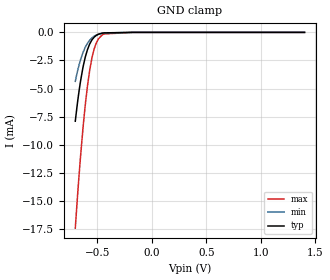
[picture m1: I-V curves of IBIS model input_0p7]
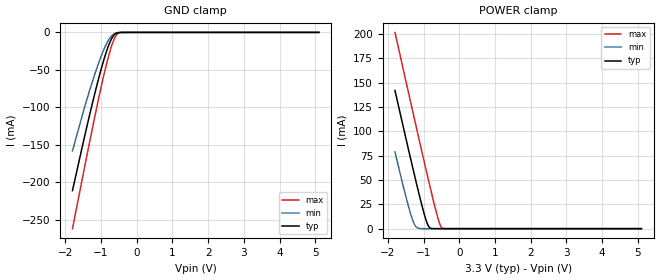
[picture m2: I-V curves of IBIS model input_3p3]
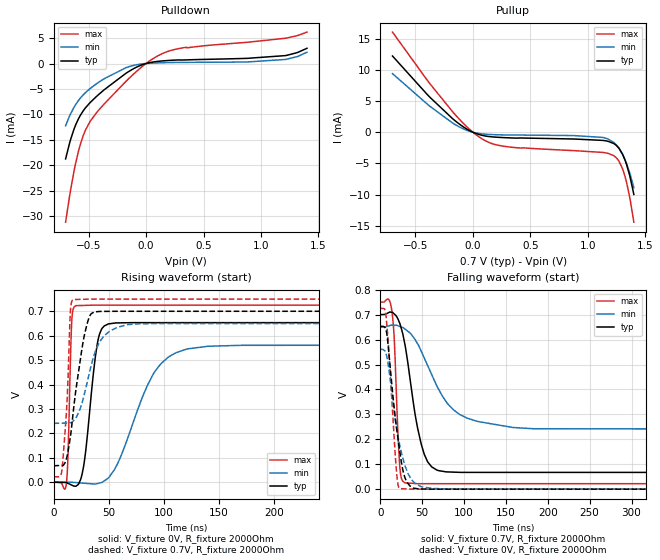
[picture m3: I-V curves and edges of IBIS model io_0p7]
|Texas Instruments Incorporated
| SN74AXCH8T245 8-Bit Dual-Supply Bus Transceiver with Configurable Voltage
| Translation, Tri-State Outputs, and Bus-Hold Circuitry
[IBIS Ver]   4.1
[File name]   sn74axch8t245.ibs
[Date]   01/24/2019
[File Rev]   2.0
[Source]
| Texas Instruments Incorporated.
| Analog-eLab Design Center, HPA
| 12500 TI Blvd
| Dallas, TX -75243
[Notes]
| Rev 2.0: 01/24/2019
| - Added SN74AXCH8T245RHL component
| Rev 1.0: 08/07/2018
| - Initial version of the model
| - Model generated from simulations in SPECTRE
| - Warnings regarding combined Non-monotonicity of various models
|   have been reviewed and considered minor and can be ignored.
| - C_comp although listed in numerical order of value are
|   obtained from varying PVT conditions. For PVT conditions for
|   each specific value refer the buffer description under
|   respective [Model]. IBIS model user is responsible for using
|   appropriate C_comp to simulate for Signal Integrity.
[Disclaimer]
| This model is designed as an aid for customers of Texas Instruments.
| TI and its licensors and suppliers make no warranties, either expressed
| or implied, with respect to this  model, including the warranties of
| merchantability or fitness for a particular purpose. The model is
| provided solely on an "as is" basis. The entire risk as to its quality
| and performance is with the customer.
| This model is subject to change without notice. Texas Instruments
| Incorporated is not responsible for updating this model.
[Copyright]
(C) Copyright 2019 Texas Instruments Incorporated.All rights reserved.
|  Component SN74AXCH8T245PW 24-pin TSSOP - PW package
|  Part # SN74AXCH8T245PW
[Component]   SN74AXCH8T245PW
[Manufacturer]  TI
[Package]   |24 TSSOP - PW package
|   typ   min   max
R_pkg   0.1143375   0.06811   0.12769
L_pkg   3.405334167nH   2.85598nH   4.17092nH
C_pkg   0.565412083pF   0.46044pF   0.71557pF
[Pin]  signal_name model_name  R_pin   L_pin   C_pin
1   VCCA   power   0.06958   3.86966nH   0.71557pF
2   DIR1   input   0.12094   3.80225nH   0.66679pF
3   A1   io   0.12769   3.54754nH   0.57242pF
4   A2   io   0.12362   3.25170nH   0.50771pF
5   A3   io   0.11601   3.02250nH   0.49462pF
6   A4   io   0.10931   2.86990nH   0.46105pF
7   A5   io   0.10845   2.85719nH   0.46044pF
8   A6   io   0.11376   2.99109nH   0.49241pF
9   A7   io   0.11998   3.20023nH   0.50408pF
10   A8   io   0.12312   3.48368nH   0.56447pF
11   DIR2   input   0.12091   3.81199nH   0.66374pF
12   GND   gnd   0.11675   4.13953nH   0.67876pF
13   GND   gnd   0.06811   3.82650nH   0.71298pF
14   B8   io   0.12091   3.81016nH   0.66711pF
15   B7   io   0.12766   3.55445nH   0.57259pF
16   B6   io   0.12359   3.25719nH   0.50787pF
17   B5   io   0.11599   3.02618nH   0.49474pF
18   B4   io   0.10929   2.87119nH   0.46118pF
19   B3   io   0.10845   2.85598nH   0.46051pF
20   B2   io   0.11377   2.98788nH   0.49236pF
21   B1   io   0.12   3.19513nH   0.50408pF
22   nOE   input   0.12314   3.47698nH   0.56494pF
23   VCCB   power   0.12375   3.84820nH   0.66804pF
24   VCCB   power   0.11932   4.17092nH   0.68143pF
|  Component SN74AXCH8T245RHL 24-pin VQFN - RHL package
|  Part # SN74AXCH8T245RHL
[Component]   SN74AXCH8T245RHL
[Manufacturer]  TI
[Package]   |24 VQFN - RHL package
|   typ   min   max
R_pkg   0.085   0.058   0.116
L_pkg   1.593n   1.101n   2.229n
C_pkg   0.258p   0.219p   0.337p
[Pin]  signal_name model_name   R_pin   L_pin   C_pin
1   VCCA   power   0.0589   1.5334n   0.3373p
2   DIR1   input   0.1148   2.1925n   0.2676p
3   A1   io   0.0984   1.7889n   0.2917p
4   A2   io   0.0841   1.4994n   0.2570p
5   A3   io   0.0723   1.2607n   0.2333p
6   A4   io   0.0655   1.1245n   0.2200p
7   A5   io   0.0637   1.1101n   0.2185p
8   A6   io   0.0688   1.2432n   0.2289p
9   A7   io   0.0788   1.4543n   0.2506p
10   A8   io   0.0925   1.7374n   0.2753p
11   DIR2   input   0.1138   2.1938n   0.2623p
12   GND   gnd   0.1074   2.0415n   0.2530p
13   GND   gnd   0.0585   1.5096n   0.3326p
14   B8   io   0.1153   2.1253n   0.2676p
15   B7   io   0.0992   1.7605n   0.2916p
16   B6   io   0.0837   1.4781n   0.2571p
17   B5   io   0.0716   1.2733n   0.2332p
18   B4   io   0.0645   1.1262n   0.2200p
19   B3   io   0.0636   1.1010n   0.2188p
20   B2   io   0.0699   1.2254n   0.2290p
21   B1   io   0.0807   1.4310n   0.2511p
22   nOE   input   0.0943   1.7202n   0.2780p
23   VCCB   power   0.1164   2.2294n   0.2692p
24   VCCB   power   0.1093   2.0732n   0.2573p
|   Model Selectors
[Model Selector] input
input_0p7   0.7V   digital Input
input_3p3   3.3V   digital Input
[Model Selector] io
io_0p7   0.7V   digital I/O
io_3p3   3.3V   digital I/O
| Models and submodels in the file (4): input_0p7 (Input), input_3p3 (Input), io_0p7 (I/O), io_3p3 (I/O)
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|   input_0p7 Model
[Model]   input_0p7
Model_type   Input
Vinl = 0.21
Vinh = 0.49
|   typ   min   max
C_comp   7.40696E-13   6.45127E-13   8.98734E-13
[Model spec]
|subparameter
Vinl   0.21   0.195   0.225
Vinh   0.49   0.455   0.525
| Where Nom  PVT is Nominal Process, 0.7V, 27C
|   Fast PVT is Strong Process,  0.75V, -40C
|   Slow PVT is Weak Process,   0.65, 130C
[Voltage Range]   0.7   0.65   0.75
|Junction Temperature
[Temperature Range]   27   130   -40
[Power Clamp Reference]   0.7   0.65   0.75
[GND Clamp Reference]   0   0   0
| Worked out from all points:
|   GND clamp passes 1 mA (typ) near -0.57 V on its own axis
[GND Clamp]
|   Voltage   I(typ)   I(min)   I(max)
-700mV    -7.896mA   -4.354mA   -17.4mA
-676.9mV  -6.033mA   -3.335mA   -14.2mA
-651.7mV  -4.329mA   -2.43mA    -11.02mA
-624.4mV  -2.873mA   -1.673mA   -7.992mA
-588.7mV  -1.545mA   -978.4uA   -4.797mA
-567.7mV  -1.026mA   -696.2uA   -3.358mA
-548.8mV  -691.6uA   -504.6uA   -2.342mA
-527.8mV  -434.7uA   -346.8uA   -1.503mA
-487.9mV  -168.3uA   -161.7uA   -574.9uA
-454.3mV  -71.1uA    -80.61uA   -230.7uA
-175mV    -4.456nA   -77.57nA   0A
1.4V      0A         0A         0A
[POWER Clamp]
|   Voltage   I(typ)   I(min)   I(max)
-700mV    0A         0A         0A
0V        0A         0A         0A
1.4V      0A         0A         0A
|   input_3p3 Model
[Model]   input_3p3
Model_type   Input
Vinl = 0.8
Vinh = 2.0
|   typ   min   max
C_comp   1.86062E-12   1.26954E-12   2.13619E-12
| Where Nom  PVT is Nominal Process, 3.3V, 27C
|   Fast PVT is Strong Process,  3.6V, -40C
|   Slow PVT is Weak Process,   3.0V, 130C
[Voltage Range]   3.3   3   3.6
|Junction Temperature
[Temperature Range]   27   130   -40
[Power Clamp Reference]   3.3   3   3.6
[GND Clamp Reference]   0   0   0
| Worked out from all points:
|   GND clamp passes 1 mA (typ) near -0.57 V on its own axis
|   POWER clamp passes 1 mA (typ) near -0.83 V on its own axis
[GND Clamp]
|   Voltage   I(typ)   I(min)   I(max)
-1.8V     -210.9mA   -157.9mA   -261.6mA
-1.49V    -144.7mA   -104.6mA   -186.5mA
-1.296V   -105.2mA   -73.69mA   -140.6mA
-1.117V   -70.54mA   -47.4mA    -99.2mA
-951.3mV  -41.37mA   -26.15mA   -63.06mA
-820.2mV  -21.52mA   -12.61mA   -37.23mA
-716.7mV  -9.415mA   -5.207mA   -19.86mA
-613.2mV  -2.39mA    -1.422mA   -6.892mA
-523.5mV  -394uA     -320.5uA   -1.365mA
-426.9mV  -33.77uA   -44.18uA   -102.3uA
-68.1mV   0A         0A         0A
5.1V      0A         0A         0A
[POWER Clamp]
|   Voltage   I(typ)   I(min)   I(max)
-1.8V     141.9mA    78.74mA    201.4mA
-1.414V   79.93mA    21.78mA    138.3mA
-1.296V   61.5mA     8.016mA    119.2mA
-1.234V   51.89mA    3.123mA    109.2mA
-1.151V   39.29mA    456.6uA    95.81mA
-985.8mV  15.65mA    4.189uA    69.3mA
-868.5mV  3.093mA    131.9nA    50.79mA
-799.5mV  400.9uA    7.757nA    40.08mA
-571.8mV  47.54nA    0A         7.669mA
-516.6mV  0A         0A         2.383mA
-468.3mV  0A         0A         390.4uA
5.1V      0A         0A         0A
|   io_0p7 Model
[Model]   io_0p7
Model_type   I/O
Polarity   Non-Inverting
Enable   Active-High
Vinl = 0.21
Vinh = 0.49
Vmeas = 0.35
Vref = 0
Cref = 2pF
Rref = 100000
|   typ   min   max
C_comp   1.59093E-12   1.45091E-12   1.76867E-12
[Model spec]
|subparameter
Vinl   0.21   0.195   0.225
Vinh   0.49   0.455   0.525
| Where Nom  PVT is Nominal Process, 0.7V, 27C
|   Fast PVT is Strong Process,  0.75V, -40C
|   Slow PVT is Weak Process,   0.65, 130C
[Voltage Range]   0.7   0.65   0.75
|Junction Temperature
[Temperature Range]   27   130   -40
[Pullup Reference]   0.7   0.65   0.75
[Pulldown Reference]   0   0   0
[Power Clamp Reference]   0.7   0.65   0.75
[GND Clamp Reference]   0   0   0
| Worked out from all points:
|   slope of the pulldown table from 0 to 0.105 V, typ, clamps not added: 245 ohm
|   slope of the pullup table from 0 to 0.105 V, typ, clamps not added: 177 ohm
|   falling waveform, V_fixture 0.7V, R_fixture 2000Ohm: 20-80 % time 18.2ns typ, 39.2ns min, 5.31ns max; typ from 0.7 V to 0.067 V
|   rising waveform, V_fixture 0V, R_fixture 2000Ohm: 20-80 % time 8.96ns typ, 29.6ns min, 2.48ns max; typ from 0 V to 0.653 V
|   rising waveform, V_fixture 0.7V, R_fixture 2000Ohm: 20-80 % time 11.3ns typ, 15.4ns min, 4.61ns max; typ from 0.067 V to 0.7 V
|   falling waveform, V_fixture 0V, R_fixture 2000Ohm: 20-80 % time 13.3ns typ, 16.4ns min, 8.05ns max; typ from 0.653 V to 0 V
[Pulldown]
|   Voltage   I(typ)   I(min)   I(max)
-700mV    -18.72mA   -12.22mA   -31.13mA
-655.9mV  -14.87mA   -9.835mA   -24.75mA
-611.8mV  -12.01mA   -8.034mA   -19.49mA
-574mV    -10.26mA   -6.853mA   -16.04mA
-525.7mV  -8.654mA   -5.68mA    -13mA
-364mV    -5.144mA   -2.978mA   -7.924mA
-175mV    -1.915mA   -824.1uA   -3.498mA
-15.4mV   -100.3uA   -29.68uA   -267.7uA
137.9mV   501.7uA    148.6uA    1.908mA
284.9mV   705.6uA    205.4uA    2.938mA
1.209V    1.548mA    790.2uA    4.951mA
1.4V      2.99mA     2.223mA    6.169mA
[Pullup]
|   Voltage   I(typ)   I(min)   I(max)
-700mV    12.24mA    9.408mA    16.08mA
-393.4mV  5.981mA    4.459mA    8.252mA
-175mV    2.144mA    1.457mA    3.25mA
-30.1mV   269.1uA    157.5uA    478.5uA
95.9mV    -562.3uA   -293.3uA   -1.24mA
343.7mV   -920.2uA   -456.7uA   -2.418mA
1.129V    -1.309mA   -829.8uA   -3.239mA
1.226V    -1.819mA   -1.649mA   -3.765mA
1.272V    -2.615mA   -2.607mA   -4.698mA
1.324V    -4.543mA   -4.459mA   -7.194mA
1.362V    -6.85mA    -6.407mA   -10.28mA
1.4V      -9.987mA   -8.898mA   -14.44mA
[Ramp]
R_load = 2000
|   typ   min   max
dV/dt_r   0.39204/8.93061e-09   0.336677/2.96083e-08   0.435114/2.47155e-09
dV/dt_f   0.379705/1.81373e-08   0.245506/3.90185e-08   0.436817/5.27495e-09
[Falling Waveform]
V_fixture = 0.7V
V_fixture_min = 0.65V
V_fixture_max = 0.75V
R_fixture = 2000Ohm
C_fixture = 0F
|   Time   V(typ)   V(min)   V(max)
0s        700mV      650mV      750mV
13.77ns   709.6mV    658.3mV    713.2mV
16.79ns   701.8mV    657.9mV    585.5mV
23.1ns    665.5mV    652.7mV    93.58mV
29.06ns   584.5mV    642.9mV    25.72mV
48.98ns   178.3mV    551.6mV    21.99mV
68.28ns   75.67mV    408.5mV    21.99mV
94.83ns   67.46mV    299.6mV    21.99mV
158.6ns   67.3mV     247.3mV    21.99mV
500ns     67.15mV    240.8mV    21.97mV
[Rising Waveform]
V_fixture = 0V
V_fixture_min = 0V
V_fixture_max = 0V
R_fixture = 2000Ohm
C_fixture = 0F
|   Time   V(typ)   V(min)   V(max)
0s        1.01uV     12.73uV    34.55nV
11.61ns   -1.797mV   -318.9uV   -7.79mV
16.45ns   -12.07mV   -457.3uV   653.7mV
20.17ns   -16.78mV   -1.685mV   722.9mV
27.54ns   73.84mV    -4.384mV   724mV
40.07ns   576.9mV    -5.434mV   725.2mV
49.4ns    647.7mV    16.34mV    725.2mV
90.12ns   653.3mV    441.4mV    725.2mV
120.2ns   653.3mV    544.6mV    725.2mV
500ns     653.4mV    561.1mV    725.2mV
[Rising Waveform]
V_fixture = 0.7V
V_fixture_min = 0.65V
V_fixture_max = 0.75V
R_fixture = 2000Ohm
C_fixture = 0F
|   Time   V(typ)   V(min)   V(max)
0s        67.15mV    240.8mV    21.97mV
7.595ns   68.55mV    241.7mV    48.46mV
12.23ns   104.9mV    242.2mV    330.8mV
15.27ns   187.1mV    243mV      699.5mV
18.03ns   294.8mV    251.2mV    748mV
27.98ns   603.1mV    361.5mV    749.2mV
37.1ns    697.4mV    525.2mV    750mV
50.53ns   699.7mV    617.4mV    750mV
77.47ns   700mV      648.6mV    750mV
500ns     700mV      650mV      750mV
[Falling Waveform]
|Gnd
V_fixture = 0V
V_fixture_min = 0V
V_fixture_max = 0V
R_fixture = 2000Ohm
C_fixture = 0F
|   Time   V(typ)   V(min)   V(max)
0s        653.4mV    561.1mV    725.2mV
6.691ns   639.4mV    544.7mV    696.1mV
9.966ns   551.2mV    485.1mV    559.9mV
18.77ns   259.8mV    256.7mV    88.59mV
20.96ns   203.9mV    213.4mV    18.95mV
23.3ns    147.2mV    173.8mV    2.08mV
28.93ns   49.97mV    98.82mV    1.338mV
35.13ns   13.3mV     49.68mV    630.3uV
63ns      68.08uV    2.704mV    15.12uV
500ns     847.1nV    12.72uV    48.33nV
